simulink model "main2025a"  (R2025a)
settings: Solver=FixedStepAuto  StartTime=0.0  StopTime=inf  FixedStep=0.1  RelTol=1e-3
undefined symbols (not defined in the file): DiscIntNeverNeededParam
libraries: simulink_extras x2, arduinolib x1

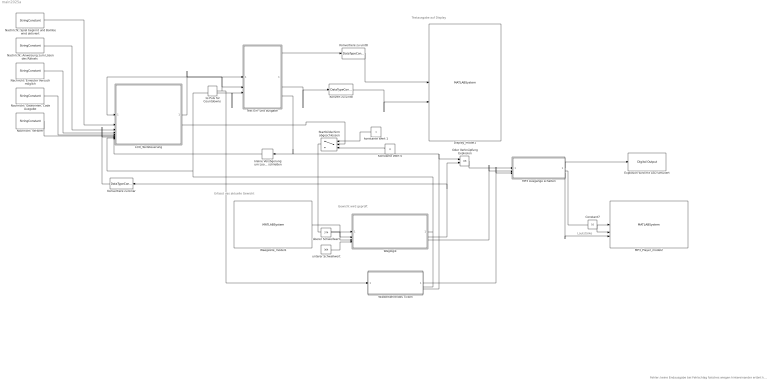
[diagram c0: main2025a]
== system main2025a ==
  note: Gewicht wird geprüft
  note: Lautstärke
  note: Erfasst das aktuelle Gewicht
  note: Textausgabe auf Display
  note: Fehler: keine Endausgabe bei Fehlschlag falsches wiegen hintereinander ertönt kein boom
  "1s Puls für Countdowns " : DiscretePulseGenerator  PulseType=Time based  Period=0.2  PulseWidth=50
  Constant7 : Constant  Value=10  OutDataTypeStr=uint8
  Display_model1 : MATLABSystem  System=Display  SampleTime=0.1
  "Explosion wird mit LED simuliert " : arduinolib/Digital Output  pinNumber=18  Direction=output  blockPlatform=arduino
  Konstante Wert 0 : Constant  Value=0
  Konvert zu uint8 : DataTypeConversion  OutDataTypeStr=uint8
  Konvertiere zu binär : DataTypeConversion  OutDataTypeStr=boolean
  Konvertiere zu uint8 : DataTypeConversion  OutDataTypeStr=uint8
  LCD_Textsteuerung : Subsystem
  MP3 Ausgänge schalten : Subsystem
  MP3_Player_model2 : MATLABSystem  System=MP3_Player  SampleTime=0.2
  "Nachricht: Anweisung zum Lösen des Rätsels " : StringConstant  String="\" Mit exakt 175ml  entschaerfst du mich!  V1=75ml, V2=125ml\""
  Nachricht: Erneuter Versuch möglich : StringConstant  String="\"Schade, aber du kannst es noch einmal versuchen !\""
  "Nachricht: Gewonnen, Code Ausgabe" : StringConstant  String="\"Herzlichen Glueckwunsch, dein Code ist        1337 !\""
  Nachricht: Spiel beginnt und Bombe wird aktiviert : StringConstant  String="\"Hallo, ich bin eine Bombe. Du hast mich gerade aktiviert !\""
  Nachricht: Verloren : StringConstant  String="\"Die Zeit hat leider nicht gereicht. Klappe den Deckel zu\""
  Oder Verknüpfung Explosion : Logic  Operator=OR  AllPortsSameDT=off  OutDataTypeStr=boolean
  Startbildschirm abgeschlossen : Switch  Criteria=u2 > Threshold  Threshold=10
  Text Ein- und ausgabe : MATLAB Function  TreatAsAtomicUnit=on
  Waegzelle_model1 : MATLABSystem  System=Waegzelle  SampleTime=0.5
  Wiederkehrendes Ticken : Subsystem
  Wäglogik : Subsystem
  kleine Verzögerung um Loop nicht zu schließen : Delay  DelayLength=1
  konstante Wert 1 : Constant
  oberer Schwellwert : Constant  Value=374
  unterer Schwellwert : Constant  Value=364
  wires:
  Constant7/1 -> MP3_Player_model2/2
  Konvert zu uint8/1 -> Display_model1/2
  Text Ein- und ausgabe/2(row_idx) -> Konvert zu uint8/1
  Konvertiere zu uint8/1 -> Display_model1/1
  Text Ein- und ausgabe/1(text_line) -> Konvertiere zu uint8/1
  "1s Puls für Countdowns "/1 -> Wiederkehrendes Ticken/1(Puls), Text Ein- und ausgabe/2(pulse_trigger), LCD_Textsteuerung/1(In Puls)
  Konstante Wert 0/1 -> Startbildschirm abgeschlossen/3
  konstante Wert 1/1 -> Startbildschirm abgeschlossen/1
  Text Ein- und ausgabe/4(timer_done) -> Wiederkehrendes Ticken/3(Rätsel abgelaufen), Oder Verknüpfung Explosion/1, kleine Verzögerung um Loop nicht zu schließen/1
  Wäglogik/1(Wagge korrektes Gewicht) -> Wiederkehrendes Ticken/2(Rätsel gelöst), LCD_Textsteuerung/8(In Stop bei Erfolg), Text Ein- und ausgabe/3(stop_signal)
  Wäglogik/2(Waage falsches Gewicht) -> Konvertiere zu binär/1, Oder Verknüpfung Explosion/2
  Konvertiere zu binär/1 -> LCD_Textsteuerung/7(In Waage falsches Gewicht)
  LCD_Textsteuerung/1(Out Display) -> Text Ein- und ausgabe/1(full_text)
  LCD_Textsteuerung/2(Out Startausgabe abgeschlossen) -> Startbildschirm abgeschlossen/2
  MP3 Ausgänge schalten/2(Out MP3 Track1) -> MP3_Player_model2/1
  MP3 Ausgänge schalten/1(Out LED Streifen1) -> "Explosion wird mit LED simuliert "/1
  MP3 Ausgänge schalten/3(Out MP3 Stop1) -> MP3_Player_model2/3
  Wäglogik/3(MP3_Ausgang unlocked) -> MP3 Ausgänge schalten/2(In Track unlocked1)
  Wiederkehrendes Ticken/1(Spiele Track 3) -> MP3 Ausgänge schalten/3(In Track Uhr1)
  Oder Verknüpfung Explosion/1 -> MP3 Ausgänge schalten/1(In Track Explosion1)
  unterer Schwellwert/1 -> Wäglogik/4(In unterer Schwellwert)
  oberer Schwellwert/1 -> Wäglogik/3(In oberer Schwellwert)
  Waegzelle_model1/1 -> Wäglogik/2(Eingang Gewicht)
  Startbildschirm abgeschlossen/1 -> Wäglogik/1(Eingang Wägprozess starten)
  Nachricht: Spiel beginnt und Bombe wird aktiviert/1 -> LCD_Textsteuerung/2(Begrünzungstext)
  kleine Verzögerung um Loop nicht zu schließen/1 -> LCD_Textsteuerung/9(In Zeit abgelaufen)
  "Nachricht: Anweisung zum Lösen des Rätsels "/1 -> LCD_Textsteuerung/3(Anweisungstext)
  Nachricht: Erneuter Versuch möglich/1 -> LCD_Textsteuerung/4(Failtext)
  "Nachricht: Gewonnen, Code Ausgabe"/1 -> LCD_Textsteuerung/5(Erfolgstext)
  Nachricht: Verloren/1 -> LCD_Textsteuerung/6(Komplett Versagt)

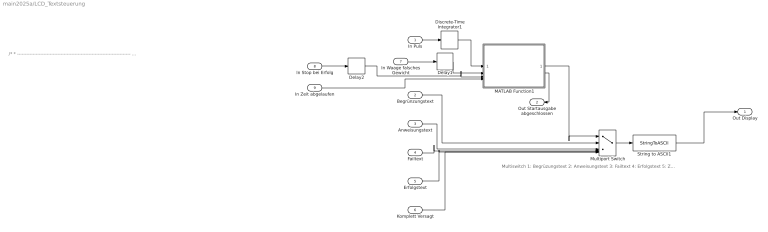
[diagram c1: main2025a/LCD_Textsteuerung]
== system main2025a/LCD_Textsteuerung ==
  note: Multiswitch 1: Begrüzungstext 2: Anweisungstext 3: Failtext 4: Erfolgstext 5: Zeit abgelaufen
  note: /* * ------------------------------------------------------------------------- * Funktion: Display Ausgänge schalten * ------------------------------------------------------------------------- * Beschreibung: Schaltet die Strings zum Displayeingang je nach Triggersignal durch * * Eingänge: * 1: In Puls [boolean] * 2: Begrüßungstext [String] * 3: Anweisungstext [String] * 4: Failtext [String] * 5: Erfolstext [String] * 6: Komplett versgt [String] * 7: In Waage falsches Gewicht [boolean] * 8: Stop bei Erfolg [boolean] * Ausgänge: * 1: Out Display [ASCII] * 2: Startausgabe abgeschlossen [boolean] * Ersteller: Tobias Brandt, Seda Ünal * Datum: 20.11.2025 * Letzte Änderung: 11.01.2026 * ------------------------------------------------------------------------- */
  In Puls : Inport
  Begrünzungstext : Inport  Port=2
  Anweisungstext : Inport  Port=3
  Failtext : Inport  Port=4
  Erfolgstext : Inport  Port=5
  Komplett Versagt : Inport  Port=6
  In Waage falsches Gewicht : Inport  Port=7
  In Stop bei Erfolg : Inport  Port=8
  In Zeit abgelaufen : Inport  Port=9
  Delay1 : Delay  DelayLength=1
  Delay2 : Delay  DelayLength=1
  Discrete-Time Integrator1 : DiscreteIntegrator  SampleTime=-1  ICPrevOutput=DiscIntNeverNeededParam  ICPrevScaledInput=DiscIntNeverNeededParam
  MATLAB Function1 : MATLAB Function  TreatAsAtomicUnit=on
  Multiport Switch : MultiPortSwitch  Inputs=5
  String to ASCII1 : StringToASCII  OutputVectorSize=82
  Out Display : Outport
  Out Startausgabe abgeschlossen : Outport  Port=2
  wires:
  Anweisungstext/1 -> Multiport Switch/3
  In Waage falsches Gewicht/1 -> Delay1/1
  Delay2/1 -> MATLAB Function1/3(stop_success)
  MATLAB Function1/1(display_out) -> Multiport Switch/1
  Begrünzungstext/1 -> Multiport Switch/2
  MATLAB Function1/2(start_done) -> Out Startausgabe abgeschlossen/1
  Komplett Versagt/1 -> Multiport Switch/6
  Failtext/1 -> Multiport Switch/4
  In Zeit abgelaufen/1 -> MATLAB Function1/4(time_out)
  Multiport Switch/1 -> String to ASCII1/1
  In Puls/1 -> Discrete-Time Integrator1/1
  In Stop bei Erfolg/1 -> Delay2/1
  String to ASCII1/1 -> Out Display/1
  Erfolgstext/1 -> Multiport Switch/5
  Delay1/1 -> MATLAB Function1/2(waage_fail)
  Discrete-Time Integrator1/1 -> MATLAB Function1/1(impuls_in)

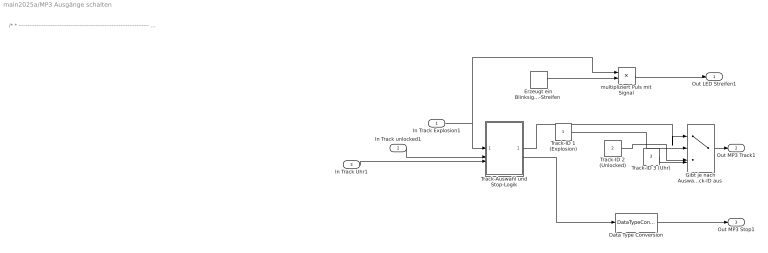
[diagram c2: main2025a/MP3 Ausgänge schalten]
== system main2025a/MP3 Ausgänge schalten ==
  note: /* * ------------------------------------------------------------------------- * Funktion: Steuerung LED und MP3-Trackauswahl * ------------------------------------------------------------------------- * Beschreibung: Wählt basierend auf drei Eingangstriggern (Explosion, * Unlocked, Uhr) die entsprechende MP3-Track-ID aus und * generiert ein Stop-Signal. Zusätzlich wird speziell für * den Fall "Explosion" ein Blinksignal für den LED-Streifen * erzeugt. * * Eingänge: * 1: In Track Explosion1 [boolean] - Trigger für Explosionseffekt * 2: In Track unlocked1 [boolean] - Trigger für "Unlocked"-Sound * 3: In Track Uhr1 [boolean] - Trigger für Uhr-Sound * * Ausgänge: * 1: Out LED Streifen1 [signal] - Blinksignal (aktiv nur bei Explosion) * 2: Out MP3 Track1 [integer] - ID des zu spielenden Tracks (1, 2 oder 3) * 3: Out MP3 Stop1 [boolean] - Steuersignal zum Stoppen des Players * * Ersteller: Tobias Brandt, Seda Ünal * Datum: 20.11.2025 * Letzte Änderung: 22.12.2025 * ------------------------------------------------------------------------- */
  In Track Explosion1 : Inport
  In Track unlocked1 : Inport  Port=2
  In Track Uhr1 : Inport  Port=3
  Data Type Conversion : DataTypeConversion  OutDataTypeStr=boolean
  "Erzeugt ein Blinksignal für den LED-Streifen " : DiscretePulseGenerator  PulseType=Time based  Period=1  PulseWidth=50
  "Gibt je nach Auswahl die passende Track-ID aus " : MultiPortSwitch  Inputs=4
  Track-Auswahl und Stop-Logik : MATLAB Function  TreatAsAtomicUnit=on
  Track-ID 1 (Explosion) : Constant  OutDataTypeStr=uint8
  Track-ID 2 (Unlocked) : Constant  Value=2  OutDataTypeStr=uint8
  Track-ID 3 (Uhr) : Constant  Value=3  OutDataTypeStr=uint8
  multipliziert Puls mit Signal : Product
  Out LED Streifen1 : Outport
  Out MP3 Track1 : Outport  Port=2
  Out MP3 Stop1 : Outport  Port=3
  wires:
  Track-ID 1 (Explosion)/1 -> "Gibt je nach Auswahl die passende Track-ID aus "/2
  Track-ID 2 (Unlocked)/1 -> "Gibt je nach Auswahl die passende Track-ID aus "/3
  Track-ID 3 (Uhr)/1 -> "Gibt je nach Auswahl die passende Track-ID aus "/4
  In Track unlocked1/1 -> Track-Auswahl und Stop-Logik/2(u2)
  In Track Uhr1/1 -> Track-Auswahl und Stop-Logik/3(u3)
  "Gibt je nach Auswahl die passende Track-ID aus "/1 -> Out MP3 Track1/1
  In Track Explosion1/1 -> multipliziert Puls mit Signal/1, Track-Auswahl und Stop-Logik/1(u1)
  multipliziert Puls mit Signal/1 -> Out LED Streifen1/1
  "Erzeugt ein Blinksignal für den LED-Streifen "/1 -> multipliziert Puls mit Signal/2
  Track-Auswahl und Stop-Logik/1(y) -> "Gibt je nach Auswahl die passende Track-ID aus "/1
  Track-Auswahl und Stop-Logik/2(stop) -> Data Type Conversion/1
  Data Type Conversion/1 -> Out MP3 Stop1/1

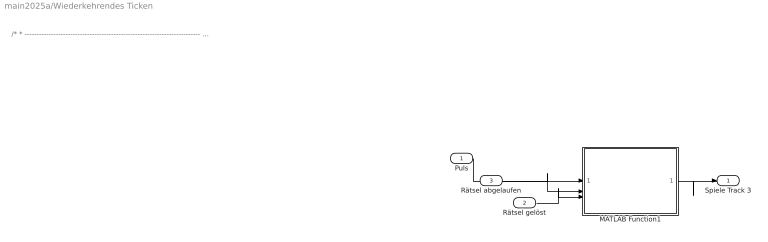
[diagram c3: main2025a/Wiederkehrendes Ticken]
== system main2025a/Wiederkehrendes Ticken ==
  note: /* * ------------------------------------------------------------------------- * Funktion: Sound-Trigger Ticken * ------------------------------------------------------------------------- * Beschreibung: Erzeugt ein Triggersignal (für Track 3/Ticken) basierend * auf einem Taktpuls, abhängig vom Status des Rätsels * (ob gelöst oder abgelaufen). * * Eingänge: * 1: Puls [boolean] * 2: Rätsel gelöst [boolean] * 3: Rätsel abgelaufen [boolean] * * Ausgänge: * 1: Spiele Track 3 [trigger/boolean] * * Ersteller: Tobias Brandt, Seda Ünal * Datum: 20.11.2025 * Letzte Änderung: 11.01.2026 * ------------------------------------------------------------------------- */
  Puls : Inport
  Rätsel gelöst : Inport  Port=2
  Rätsel abgelaufen : Inport  Port=3
  MATLAB Function1 : MATLAB Function  TreatAsAtomicUnit=on
  Spiele Track 3 : Outport
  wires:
  MATLAB Function1/1(display_out) -> Spiele Track 3/1
  Puls/1 -> MATLAB Function1/1(impuls_in)
  Rätsel gelöst/1 -> MATLAB Function1/3(stop_success)
  Rätsel abgelaufen/1 -> MATLAB Function1/2(waage_fail)

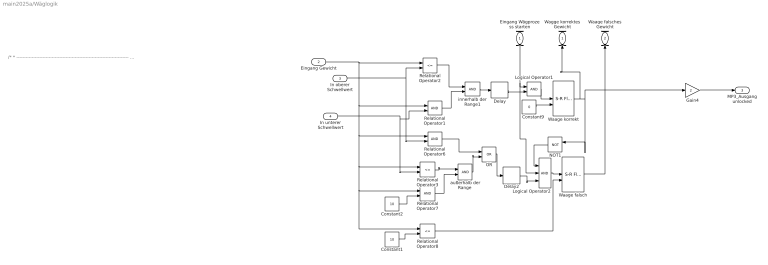
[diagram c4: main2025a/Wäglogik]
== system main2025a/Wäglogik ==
  note: /* * ------------------------------------------------------------------------- * Funktion: Waagen-Steuerungslogik und Gewichtsprüfung * ------------------------------------------------------------------------- * Beschreibung: Überprüft, ob ein gemessenes Gewicht nach einem Startsignal * für eine definierte Zeit stabil innerhalb oder außerhalb * vorgegebener Schwellwerte liegt. Setzt entsprechende * Status- und Steuersignale. * * Eingänge: * 1: Eingang Wägprozess starten [boolean] - Trigger für den Vorgang * 2: Eingang Gewicht [uint8] - Aktueller Messwert der Waage * 3: oberer Schwellwert [uint8] - Obere Grenze für korrektes Gewicht * 4: unterer Schwellwert [uint8] - Untere Grenze für korrektes Gewicht * * Ausgänge: * 1: Waage korrektes Gewicht [boolean] - Status "Gewicht OK" * 2: Waage falsches Gewicht [boolean] - Status "Gewicht nicht OK" * 3: MP3_Ausgang unlocked [uint8] - Steuersignal für MP3 (basiert auf "Waage korrekt") * * Ersteller: Tobias Brandt, Seda Ünal * Datum: 20.11.2025 * Letzte Änderung: 11.01.2026 * ------------------------------------------------------------------------- */
  Eingang Wägprozess starten : Inport
  Eingang Gewicht : Inport  Port=2
  In oberer Schwellwert : Inport  Port=3
  In unterer Schwellwert : Inport  Port=4
  Constant1 : Constant  Value=10
  Constant2 : Constant  Value=10
  Constant9 : Constant  Value=0  OutDataTypeStr=boolean
  Delay : Delay
  Delay2 : Delay  DelayLength=3
  Gain4 : Gain  Gain=2
  Logical Operator1 : Logic  AllPortsSameDT=off  OutDataTypeStr=boolean
  Logical Operator2 : Logic  Inputs=3  AllPortsSameDT=off  OutDataTypeStr=boolean
  NOT1 : Logic  Operator=NOT  IconShape=distinctive  AllPortsSameDT=off  OutDataTypeStr=boolean
  OR : Logic  Operator=OR  IconShape=distinctive  AllPortsSameDT=off  OutDataTypeStr=boolean
  Relational Operator1 : RelationalOperator  OutDataTypeStr=boolean  RndMeth=Simplest
  Relational Operator2 : RelationalOperator  Operator=<=  OutDataTypeStr=boolean  RndMeth=Simplest
  Relational Operator3 : RelationalOperator  Operator=<=  OutDataTypeStr=boolean  RndMeth=Simplest
  Relational Operator6 : RelationalOperator  OutDataTypeStr=boolean  RndMeth=Simplest
  Relational Operator7 : RelationalOperator  OutDataTypeStr=boolean  RndMeth=Simplest
  Relational Operator8 : RelationalOperator  Operator=<=  OutDataTypeStr=boolean  RndMeth=Simplest
  Waage falsch : simulink_extras/Flip Flops/S-R Flip-Flop  initial_condition=0
  Waage korrekt : simulink_extras/Flip Flops/S-R Flip-Flop  initial_condition=0
  "außerhalb der Range " : Logic  AllPortsSameDT=off  OutDataTypeStr=boolean
  innerhalb der Range1 : Logic  AllPortsSameDT=off  OutDataTypeStr=boolean
  Wagge korrektes Gewicht : Outport
  Waage falsches Gewicht : Outport  Port=2
  MP3_Ausgang unlocked : Outport  Port=3
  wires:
  Waage korrekt/1 -> Wagge korrektes Gewicht/1, Gain4/1, NOT1/1
  NOT1/1 -> Logical Operator2/1
  Relational Operator6/1 -> OR/1
  Logical Operator2/1 -> Waage falsch/1
  "außerhalb der Range "/1 -> OR/2
  Relational Operator1/1 -> innerhalb der Range1/2
  Constant2/1 -> Relational Operator7/2
  OR/1 -> Delay2/1
  Waage falsch/1 -> Waage falsches Gewicht/1
  Relational Operator8/1 -> Waage falsch/2
  innerhalb der Range1/1 -> Delay/1
  Delay/1 -> Logical Operator1/2
  In oberer Schwellwert/1 -> Relational Operator6/2, Relational Operator2/2
  Logical Operator1/1 -> Waage korrekt/1
  Gain4/1 -> MP3_Ausgang unlocked/1
  Delay2/1 -> Logical Operator2/3
  Relational Operator2/1 -> innerhalb der Range1/1
  Eingang Wägprozess starten/1 -> Logical Operator2/2, Logical Operator1/1
  Relational Operator3/1 -> "außerhalb der Range "/1
  Eingang Gewicht/1 -> Relational Operator2/1, Relational Operator8/1, Relational Operator7/1, Relational Operator3/1, Relational Operator6/1, Relational Operator1/1
  In unterer Schwellwert/1 -> Relational Operator3/2, Relational Operator1/2
  Constant9/1 -> Waage korrekt/2
  Relational Operator7/1 -> "außerhalb der Range "/2
  Constant1/1 -> Relational Operator8/2

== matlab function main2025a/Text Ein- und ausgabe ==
function [text_line, row_idx, write_enable, timer_done] = Displayausgabe(full_text, pulse_trigger, stop_signal)
% FUNKTION: Displayausgabe
%
% BESCHREIBUNG:
%   Diese Funktion steuert ein 4x20 LCD-Display in zwei Phasen:
%   1. Schreibmaschinen-Modus: Der Text wird Zeichen für Zeichen aufgebaut.
%   2. Info-Modus: Nach Abschluss des Textes rotiert die Anzeige durch die 
%      Textzeilen und zeigt anschließend einen Countdown-Timer an.
%
% ERSTELLUNGSDATUM:       30.11.2025
% LETZTES ÄNDERUNGSDATUM: 22.12.2025
%
% EINGÄNGE:
%   full_text     - (String/Array) Der anzuzeigende Gesamttext
%   pulse_trigger - (Boolean) Taktflanke, die die Logik weiterschaltet 
%   stop_signal   - (Int/Bool) Wenn 1, wird der Timer angehalten 
%
% AUSGÄNGE:
%   text_line     - (uint8 [20x1]) Die aktuelle Zeile für das Display (ASCII)
%   row_idx       - (uint8) Die Zeilennummer (0 bis 3), die beschrieben werden soll
%   write_enable  - (uint8) Flag, das dem Display sagt "Jetzt schreiben" 
%   timer_done    - (uint8) Flag: 1 wenn der Timer 0 erreicht hat, sonst 0
% ----------------------------------------------------------------------------------

% -- 1. Persistente Variablen definieren --
persistent cursor timer_sec active_timer text_done tick_counter timer_finished_mem display_cycle;

% -- 2. Initialisierung (nur beim ersten Aufruf) --
if isempty(cursor)
    cursor = int32(1);              % Startposition des Cursors (1-basiert) für den Schreibmaschinen-Effekt
    timer_sec = int32(300);         % Startwert des Timers in Sekunden (300s = 5 Minuten)
    active_timer = false;           % Der Timer ist zu Beginn inaktiv (startet erst nach Textende)
    text_done = false;              % Flag: Tecxt wurde noh nicht vollständig "getippt"
    tick_counter = int32(0);        % Zähler für die Anzeigerotation im Info-Modus
    timer_finished_mem = false;     % Speicher für den Status "Timer abgelaufen"
    display_cycle = int32(0);       % Variable für Zyklus-Management
end

% Länge des übergebenen Textes ermitteln
len_text = int32(numel(full_text)); % Gesamtzahl der Zeichen im Text ermitteln und in int32 konvertieren

% -- 3. Zustands-Logik (wird nur bei Trigger-Impuls ausgeführt) --
if pulse_trigger
    
    % -- Phase 1: Schreibmaschinen-Effekt --
    % Solange der Text noch nicht vollständig angezeigt wurde:
    if ~text_done
        if cursor < len_text
            cursor = cursor + 1;    % Cursor eins weiter schieben (nächstes Zeichen aufdecken)
        else
            % Text ist am Ende angekommen
            text_done = true;       % Modus-Wechsel markieren
            active_timer = true;    % Timer-Logik scharfschalten
            tick_counter = int32(0);% Zähler zurücksetzen für sauberen Start von Phase 2
        end
    end
    
    % -- Phase 2: Timer & Rotation (nach Textende) --
    if text_done
        % Der Tick-Counter steuert, welche Zeile gerade angezeigt wird.
        tick_counter = tick_counter + 1; 
        
        % Zyklus dauert 5 Ticks (0, 1, 2 zeigen Text; 3, 4 zeigen Timer)
        if tick_counter >= 5
            
            % Timer-Logik: Nur einmal pro Zyklus (alle 5 Ticks) aktualisieren
            if active_timer
                if timer_sec > 0
                    if stop_signal == 0
                        % Zeit herunterzählen, wenn kein Stop-Signal anliegt
                        timer_sec = timer_sec - int32(1);
                    end
                else
                    % Zeit ist abgelaufen
                    timer_finished_mem = true;
                    active_timer = false;
                end
            end
            
            % Counter zurücksetzen, damit der Zyklus von vorn beginnt
            tick_counter = int32(0); 
        end
    end
end

% Ausgang für Timer-Status setzen 
timer_done = uint8(timer_finished_mem);


% -- 4. Ausgabe-Aufbereitung (Erstellung von text_line) --

% Leere Zeile vorbereiten (mit ASCII 32 = Leerzeichen füllen)
text_line = uint8(32 * ones(20, 1)); 

if ~text_done
    %% -- Modus A: Schreibmaschinen-Ausgabe --
    
    % Berechnen, in welcher Zeile (0-3) sich der Cursor gerade befindet
    current_row_dbl = floor(double(cursor - 1) / 20);
    row_idx = uint8(current_row_dbl);
    
    % Startindex des Textes für diese spezifische Zeile berechnen
    start_of_row = int32(current_row_dbl * 20 + 1);
    
    % Berechnen, wie viele Zeichen in dieser Zeile schon "getippt" sind
    chars_in_this_row = cursor - (start_of_row - 1);
    
    % Begrenzung auf maximal 20 Zeichen pro Zeile (Displaybreite)
    if chars_in_this_row > 20
        chars_in_this_row = int32(20);
    end
    
    % Zeichen aus dem full_text in den Ausgabe-Vektor kopieren
    if chars_in_this_row > 0
        for k = 1:chars_in_this_row
            char_pos = start_of_row + k - 1; % Position im Gesamttext
            if char_pos <= len_text
                text_line(k) = uint8(full_text(char_pos)); % ASCII-Code übernehmen
            end
        end
    end

else
    %% -- Modus B: Rotations-Ausgabe (Synchronisiert) --
    % Logik der Anzeige-Rotation basierend auf tick_counter:
    % Tick 0 -> Zeigt Zeile 0 des Textes
    % Tick 1 -> Zeigt Zeile 1 des Textes
    % Tick 2 -> Zeigt Zeile 2 des Textes
    % Tick 3 & 4 -> Zeigt Zeile 3 (den Timer)
    
    if tick_counter <= 2
        current_show_row = tick_counter; % Textzeilen 0, 1 oder 2
    else
        current_show_row = int32(3);     % Zeile 3 (Timer-Anzeige)
    end
    
    row_idx = uint8(current_show_row);   % Ausgangsvariable setzen
    
    if current_show_row < 3
        % -- Statischen Text anzeigen (Zeilen 0-2) --
        start_idx = int32(current_show_row * 20 + 1); % Startindex im Text-Array
        
        for k = 1:20
            idx = start_idx + k - 1;
            if idx <= len_text
                text_line(k) = uint8(full_text(idx)); % Zeichen kopieren
            else
                text_line(k) = uint8(32);             % Mit Leerzeichen auffüllen, falls Text kürzer
            end
        end
    else
        % -- Timer anzeigen (Zeile 3) --
        row_idx = uint8(3); 
        
        % Minuten und Sekunden berechnen
        minutes = int32(floor(double(timer_sec) / 60));
        seconds = int32(mod(double(timer_sec), 60));
        
        % String für Timer bauen: "MM:SS"
        timer_str = uint8(32 * ones(5, 1)); % Platzhalter für 5 Zeichen
        
        % ASCII-Berechnung: '0' (Wert 48) + Ziffer
        timer_str(1) = uint8('0') + uint8(floor(double(minutes)/10)); % Zehner-Minute
        timer_str(2) = uint8('0') + uint8(mod(double(minutes),10));   % Einer-Minute
        timer_str(3) = uint8(':');                                    % Doppelpunkt
        timer_str(4) = uint8('0') + uint8(floor(double(seconds)/10)); % Zehner-Sekunde
        timer_str(5) = uint8('0') + uint8(mod(double(seconds),10));   % Einer-Sekunde
        
        % Timer mittig in die Zeile schreiben (Position 8 bis 12)
        text_line(8:12) = timer_str; 
    end
end

% -- 5. Schreib-Signal --
write_enable = uint8(1); % Signalisiert dem Display-Treiber, dass Daten gültig sind

end

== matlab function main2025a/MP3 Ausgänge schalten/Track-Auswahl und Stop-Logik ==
% FUNKTION: Track-Auswahl und Stop-Logik
%
% BESCHREIBUNG:
%   Diese Funktion wählt basierend auf drei Eingangstriggern die entsprechende
%   MP3-Track-ID aus. Dabei wird eine Priorisierung angewendet 
%   (Explosion > Unlocked > Uhr). 
%   Ein interner Timer (State Machine) sorgt für die Haltezeit der Signale 
%   und generiert das Stop-Signal, wenn kein Track aktiv ist.
%
% ERSTELLUNGSDATUM:       20.11.2025
% LETZTES ÄNDERUNGSDATUM: 22.12.2025
% AUTOR:                  Tobias Brandt, Seda Ünal
%
% EINGÄNGE:
%   u1 - (bolean) Trigger Explosion (Priorität 1, reagiert auf Flanke)
%   u2 - (bolean) Trigger Unlocked (Priorität 2, reagiert auf Flanke)
%   u3 - (bolean) Signal Uhr/Ticken (Priorität 3, reagiert auf Pegel)
%
% AUSGÄNGE:
%   y    - (Integer) Aktive Track-ID (1=Explosion, 2=Unlocked, 3=Uhr, 0=Keine)
%   stop - (Boolean) Stop-Signal für den MP3-Player (1=Stop, 0=Play)
% ----------------------------------------------------------------------------------

function [y, stop] = fcn(u1, u2, u3)
    %% 1. --Eingangskonvertierung--
    u1_d = double(u1);
    u2_d = double(u2);
    u3_d = double(u3);
    
    %% 2. --Zustände merken--
    % timer_active: Zählt runter, wie lange ein Track noch anliegen soll
    % active_track: Merkt sich, welcher Track gerade spielt
    persistent u1_alt u2_alt timer_active active_track
    
    if isempty(u1_alt)
        u1_alt = 0; u2_alt = 0;
        timer_active = 0;
        active_track = 0;
    end
    
    %% 3. --Eingänge Prüfen-- (Priorität: Explosion > Lösen > Uhr)
    
    % 1. Explosion (startet nur bei 0->1 Übergang)
    if (u1_d > 0) && (u1_alt <= 0)
        active_track = 1;
        timer_active = 5; % Signal für 5 Ticks halten
    end
    
    % 2. Unlocked (Flankenerkennung, nur wenn Explosion nicht aktiv gestartet wurde)
    if (u2_d > 0) && (u2_alt <= 0) && (active_track ~= 1)
        active_track = 2;
        timer_active = 5; % Signal für 5 Ticks halten
    end
    
    % 3. Uhr (Pegelerkennung)
    % Wenn Uhr kommt und gerade nichts Wichtigeres läuft (Timer 0)
    if (u3_d > 0) && (timer_active == 0)
        active_track = 3;
        timer_active = 1; 
    end
    
    %% 4. --Ausgabe Logik--
    
    if timer_active > 0
        y = active_track;       % Den gespeicherten Track ausgeben
        stop = 0;               % Spielen erlauben!
        
        % Timer runterzählen
        timer_active = timer_active - 1; 
    else
        y = 0;
        active_track = 0;       % Reset
        stop = 1;               % Jetzt erst Stop senden
    end
    
    %% 5. --Zustand speichern--
    u1_alt = u1_d;
    u2_alt = u2_d;
end

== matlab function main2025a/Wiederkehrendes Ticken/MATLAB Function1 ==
function [display_out, start_done] = fcn(impuls_in, waage_fail, stop_success, time_out)
% FUNKTION: Display-Steuerung und Verriegelung
%
% BESCHREIBUNG:
%   Diese Funktion steuert die Statusausgabe eines Displays. Sie verriegelt den
%   Startzustand, sobald ein Impulsschwellenwert (>8) erreicht wurde.
%   Anschließend wird ein Prioritäten-basierter Statuscode (display_out) 
%   ausgegeben, der zwischen Normalbetrieb, Fehlern, Erfolg und Timeout unterscheidet.
%
% EINGÄNGE:
%   impuls_in    - (Integer) Externer Zählerstand der Impulse.
%   waage_fail   - (Boolean)  wenn die Waage falsch belegt ist.
%   stop_success - (Boolean)  wenn das Spiel erfolgreich beendet wurde.
%   time_out     - (Boolean)  wenn die Spielzeit abgelaufen ist.
%
% AUSGÄNGE:
%   display_out  - (Integer) Statuscode: 1=Warten, 2=Läuft, 3=Fehler, 4=Erfolg, 5=Timeout.
%   start_done   - (Boolean) Rückmeldung: 1 wenn das Spiel bereits gestartet wurde.
% ---------------------------------------------------------------

    % Persistent Variable: Speichert den Startzustand dauerhaft 
    persistent is_started
    
    % Initialisierung der persistenten Variable beim ersten Aufruf
    if isempty(is_started)
        is_started = 0;
    end
    
    % --- 1. START-LOGIK ---
    % Sobald die Impulse einmalig den Wert 8 überschreiten, wird das Spiel 
    % dauerhaft als gestartet markiert.
    if impuls_in > 8
        is_started = 1;
    end
    
    % Rückgabe des Startstatus an den Ausgang
    start_done = is_started;
    
    % --- 2. DISPLAY-LOGIK (Priorisierung) ---
    
    if is_started == 0
        % Zustand: Startphase / Warten auf Impulse
        display_out = 1;
        
    else
        % Zustand: Spiel ist aktiv. Die Ausgabe folgt einer Prioritätenliste.
        
        if time_out == 1
            % Höchste Priorität: Zeit abgelaufen
            display_out = 5;
            
        elseif stop_success == 1
            % Zweite Priorität: Erfolg erreicht
            display_out = 4;
            
        elseif waage_fail == 1
            % Dritte Priorität: Fehlerzustand (Waage)
            display_out = 3;
            
        else
            % Niedrigste Priorität: Regulärer Spielbetrieb
            display_out = 2;
        end
    end
end

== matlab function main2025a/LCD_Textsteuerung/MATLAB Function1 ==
function [display_out, start_done] = fcn(impuls_in, waage_fail, stop_success, time_out)
% FCN - Steuert die Anzeige-Logik und den Spielstatus basierend auf Sensordaten.
%
% Syntax:
%   [display_out, start_done] = fcn(impuls_in, waage_fail, stop_success, time_out)
%
% Beschreibung:
%   Die Funktion überwacht einen Impulszähler, um das Spiel zu starten (Latching).
%   Sobald das Spiel läuft, wird ein Status-Code (display_out) basierend auf 
%   einer festen Prioritätenliste ausgegeben.
%
% Eingabeparameter:
%   impuls_in    - Aktueller Zählerstand der Impulse (Externer Trigger)
%   waage_fail   - Flag (0/1): Fehlerzustand der Waage
%   stop_success - Flag (0/1): Erfolgreiches Beenden des Spiels
%   time_out     - Flag (0/1): Zeitlimit überschritten
%
% Ausgabeparameter:
%   display_out  - Statuscode für die Anzeige:
%                  1: Startphase / Warteposition
%                  2: Normalbetrieb (Spiel läuft)
%                  3: Fehler (Waage)
%                  4: Erfolg (Ziel erreicht)
%                  5: Timeout (Zeit abgelaufen)
%   start_done   - Flag (0/1): Gibt an, ob der Startimpuls (>8) bereits erfolgt ist
%

    % Persistent Variable: Speichert den Zustand über mehrere Aufrufe hinweg (Latching)
    persistent is_started
    
    % Initialisierung beim ersten Aufruf
    if isempty(is_started)
        is_started = 0;
    end
    
    % ---------------------------------------------------------
    % 1. START-LOGIK (Verriegelung)
    % ---------------------------------------------------------
    % Das Spiel gilt als gestartet, sobald impuls_in den Schwellenwert von 8 überschreitet.
    % Einmal gesetzt, bleibt is_started auf 1 (Latching-Verhalten).
    if impuls_in > 8
        is_started = 1;
    end
    
    % Rückmeldung, ob die Startbedingung erfüllt wurde
    start_done = is_started;
    
    % ---------------------------------------------------------
    % 2. DISPLAY-LOGIK (Zustandssteuerung)
    % ---------------------------------------------------------
    
    if is_started == 0
        % ZUSTAND A: Wartephase
        % Das Spiel wurde noch nicht durch ausreichend Impulse aktiviert.
        display_out = 1; 
        
    else
        % ZUSTAND B: Aktivphase
        % Das Spiel läuft. Die Anzeige wird durch Ereignisse mit folgender 
        % Priorität gesteuert:
        
        if time_out == 1
            % Höchste Priorität: Zeit abgelaufen
            display_out = 5;
            
        elseif stop_success == 1
            % Zweite Priorität: Erfolgreicher Abschluss
            display_out = 4;
            
        elseif waage_fail == 1
            % Dritte Priorität: Fehler an der Waage
            display_out = 3;
            
        else
            % Standardzustand: Spiel läuft ohne besondere Ereignisse
            display_out = 2;
        end
    end
end
